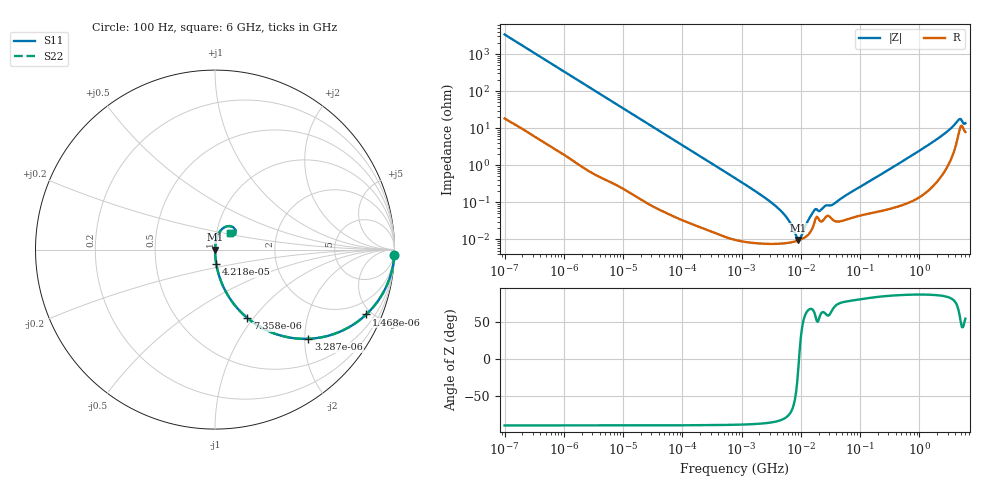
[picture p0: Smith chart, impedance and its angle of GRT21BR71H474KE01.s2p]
!Murata Part Number: GRT21BR71H474KE01
!These Parameters are Measured in Series Mode Connection
!Data Generated on Jun 19, 2026
!  o--ll--o
!Port1  Port2
!  o------o
!Operation Temp=25[degC], DC Bias Voltage=0[V]
!Freq. Start=100[Hz] Stop=6[GHz] 401[Steps]
# Hz S RI R 50
!Freq.(Hz) S11(Real) S11(Imag) S21(Real) S21(Imag) S12(Real) S12(Imag) S22(Real) S22(Imag)
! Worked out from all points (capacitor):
!   401 points, 100 Hz to 6 GHz, reference 50 ohm
!   read as one part in series: C = 469 nF near 109 Hz
!   lowest |Z| = 9.55 mohm at 9.09 MHz (marker M1)
!   series resonance near 9.331 MHz, so ESL is about 620 pH
!   S11 on the Smith chart (normalised r, x): 100 Hz: 1, -68; 1.468 kHz: 1.03, -4.66; 3.287 kHz: 1.01, -2.09; 7.358 kHz: 1.01, -0.93; 42.18 kHz: 1.00, -0.16; 6 GHz: 1.16, +0.22
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100  0.999 -0.0295  0.00103 0.0295  0.00103 0.0295  0.999 -0.0295
438  0.983 -0.1265  0.017 0.1265  0.017 0.1265  0.983 -0.1265
1468  0.843 -0.3611  0.157 0.3611  0.157 0.3611  0.843 -0.3611
2008  0.7427 -0.4345  0.2573 0.4345  0.2573 0.4345  0.7427 -0.4345
3287  0.5208 -0.4968  0.4792 0.4968  0.4792 0.4968  0.5208 -0.4968
7358  0.1807 -0.3815  0.8193 0.3815  0.8193 0.3815  0.1807 -0.3815
14402  0.0556 -0.2257  0.9444 0.2257  0.9444 0.2257  0.0556 -0.2257
40335  0.00793 -0.0851  0.9921 0.0851  0.9921 0.0851  0.00793 -0.0851
42182  0.00729 -0.0814  0.9927 0.0814  0.9927 0.0814  0.00729 -0.0814
774597  0.000117 -0.00451  0.9999 0.00451  0.9999 0.00451  0.000117 -0.00451
4246196  7.65e-05 -0.000662  0.9999 0.000662  0.9999 0.000662  7.65e-05 -0.000662
6075234  8.04e-05 -0.000338  0.9999 0.000338  0.9999 0.000338  8.04e-05 -0.000338
9090158  9.33e-05 -2.02e-05  0.9999 2.02e-05  0.9999 2.02e-05  9.33e-05 -2.02e-05
9941735  9.86e-05 4.98e-05  0.9999 -4.98e-05  0.9999 -4.98e-05  9.86e-05 4.98e-05
1.555665e7  0.000194 0.000458  0.9998 -0.000458  0.9998 -0.000458  0.000194 0.000458
1.779312e7  0.000362 0.00055  0.9996 -0.00055  0.9996 -0.00055  0.000362 0.00055
2.128304e7  0.000307 0.000513  0.9997 -0.000513  0.9997 -0.000513  0.000307 0.000513
3.482834e7  0.000336 0.000805  0.9997 -0.000805  0.9997 -0.000805  0.000336 0.000805
3.124326e8  0.000718 0.00773  0.9993 -0.00773  0.9993 -0.00773  0.000718 0.00773
1.95892e9  0.0059 0.0493  0.9941 -0.0493  0.9941 -0.0493  0.0059 0.0493
4.586474e9  0.0821 0.1313  0.9179 -0.1313  0.9179 -0.1313  0.0821 0.1313
6e9  0.0832 0.0938  0.9168 -0.0938  0.9168 -0.0938  0.0832 0.0938
